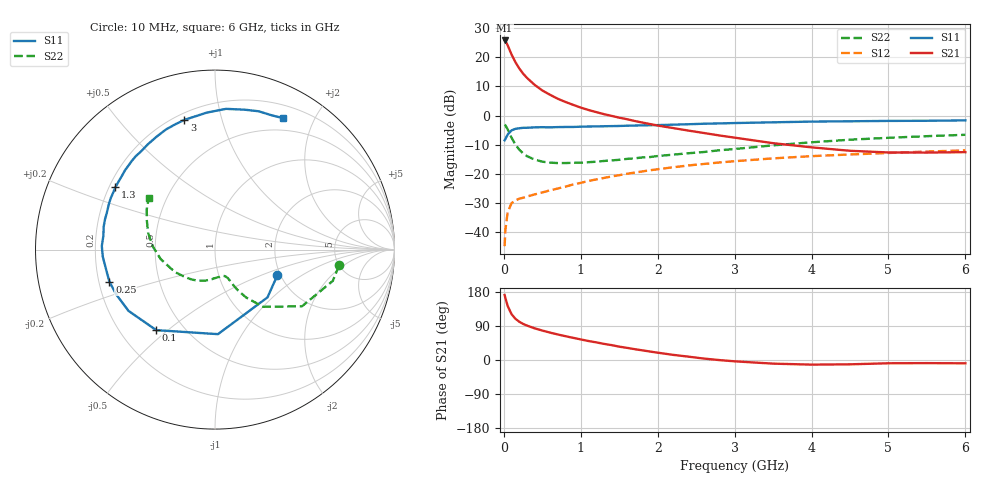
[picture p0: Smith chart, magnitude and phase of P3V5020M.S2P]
! SIEMENS Small Signal Semiconductors
! BFP181
! Si NPN RF Bipolar Junction Transistor in SOT143
! VCE = 0.5 V  IC = 20 mA
! Common Emitter S-Parameters:  March  1996
# GHz  S  MA  R  50
!  f  S11  S21  S12  S22
! GHz  MAG  ANG  MAG  ANG  MAG  ANG  MAG  ANG
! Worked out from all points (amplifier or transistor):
!   36 points, 10 MHz to 6 GHz, reference 50 ohm
!   highest |S21| = 25.8 dB at 10 MHz (marker M1)
!   |S21| within 3 dB of that: start of sweep to 71.13 MHz
!   unconditionally stable (mu >= 1): start of sweep to 25.81 MHz; 155.6 MHz to end of sweep
!   at 250 MHz: K = 1.42, MAG = 17.5 dB, |S12| = -28.2 dB
!   at 1.4 GHz: K = 3.07, MAG = 2.7 dB, |S12| = -20.9 dB
!   at 6 GHz: K = 2.47, MAG = -7.1 dB, |S12| = -12.0 dB
!   S11 on the Smith chart (normalised r, x): 10 MHz: 1.92, -0.64; 100 MHz: 0.35, -0.46; 250 MHz: 0.24, -0.14; 1.3 GHz: 0.23, +0.27; 3 GHz: 0.24, +0.76; 6 GHz: 0.35, +1.59
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0.01  0.3757 -22.4  19.48 171.7  0.0057 69.2  0.6968 -7.3
0.02  0.3955 -42.3  19.01 163.6  0.0109 67.2  0.679 -14.9
0.05  0.4714 -88.0  16.06 142.5  0.0219 55.6  0.5785 -33.1
0.1  0.5554 -126.1  11.19 120.9  0.0312 41.2  0.4166 -49.9
0.15  0.5907 -144.7  8.278 108.9  0.0349 35.9  0.3181 -57.0
0.2  0.6043 -155.5  6.454 101.0  0.0372 33.9  0.2596 -60.7
0.25  0.6148 -163.0  5.257 95.3  0.0387 33.1  0.2239 -62.7
0.3  0.6158 -168.3  4.443 90.9  0.0406 34.3  0.2008 -63.7
0.4  0.6265 -176.4  3.366 83.6  0.0441 36.6  0.1749 -65.7
0.5  0.6309 178.2  2.696 77.7  0.0477 38.6  0.1613 -68.3
0.6  0.6267 172.9  2.274 72.3  0.0519 40.9  0.1551 -71.1
0.7  0.6331 168.5  1.944 67.4  0.0557 42.9  0.1526 -73.6
0.9  0.6365 161.3  1.527 58.5  0.0653 45.4  0.1543 -80.8
1.1  0.6478 153.8  1.245 50.1  0.0751 46.7  0.1579 -88.6
1.3  0.6547 147.9  1.057 42.6  0.0846 46.8  0.1657 -96.0
1.7  0.6728 135.4  0.806 28.6  0.1046 45.9  0.184 -110.1
2.2  0.6964 122.3  0.609 13.6  0.1291 42.2  0.2128 -129.1
3  0.7426 103.3  0.417 -3.5  0.1641 34.4  0.2659 -156.2
3.5  0.7647 93.4  0.335 -9.6  0.1837 29.2  0.3075 -170.2
4.5  0.7969 78.0  0.248 -11.4  0.2143 18.4  0.3845 165.8
5.5  0.8125 66.9  0.231 -8.3  0.2408 9.0  0.442 149.3
6  0.8252 62.5  0.235 -8.7  0.2517 4.0  0.4669 142.3
